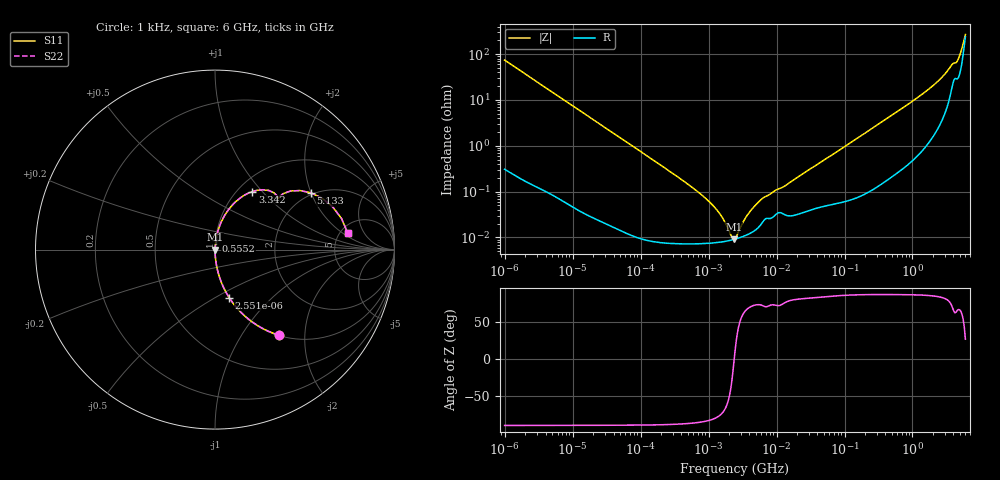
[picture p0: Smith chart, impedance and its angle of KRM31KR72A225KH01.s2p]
!Murata Part Number: KRM31KR72A225KH01
!These Parameters are Measured in Series Mode Connection
!Data Generated on Jan 08, 2026
!  o--ll--o
!Port1  Port2
!  o------o
!Operation Temp=25[degC], DC Bias Voltage=0[V]
!Freq. Start=1000[Hz] Stop=6[GHz] 401[Steps]
# Hz S RI R 50
!Freq.(Hz) S11(Real) S11(Imag) S21(Real) S21(Imag) S12(Real) S12(Imag) S22(Real) S22(Imag)
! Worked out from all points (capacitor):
!   401 points, 1 kHz to 6 GHz, reference 50 ohm
!   read as one part in series: C = 2.15 uF near 1.081 kHz
!   lowest |Z| = 9.07 mohm at 2.356 MHz (marker M1)
!   series resonance near 2.384 MHz, so ESL is about 2.1 nH
!   S11 on the Smith chart (normalised r, x): 1 kHz: 1.01, -1.48; 2.551 kHz: 1.00, -0.58; 555.2 MHz: 1.00, +0.10; 3.342 GHz: 1.17, +0.89; 5.133 GHz: 1.94, +1.99; 6 GHz: 5.78, +2.44
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1000  0.3549 -0.4764  0.6451 0.4764  0.6451 0.4764  0.3549 -0.4764
2551  0.0792 -0.2677  0.9208 0.2677  0.9208 0.2677  0.0792 -0.2677
5567  0.0183 -0.1312  0.9817 0.1312  0.9817 0.1312  0.0183 -0.1312
13657  0.00333 -0.0545  0.9967 0.0545  0.9967 0.0545  0.00333 -0.0545
186501  9.38e-05 -0.00401  0.9999 0.00401  0.9999 0.00401  9.38e-05 -0.00401
556098  7.39e-05 -0.00128  0.9999 0.00128  0.9999 0.00128  7.39e-05 -0.00128
1038191  7.51e-05 -0.000586  0.9999 0.000586  0.9999 0.000586  7.51e-05 -0.000586
1474979  7.89e-05 -0.000313  0.9999 0.000313  0.9999 0.000313  7.89e-05 -0.000313
2095531  8.66e-05 -8.08e-05  0.9999 8.08e-05  0.9999 8.08e-05  8.66e-05 -8.08e-05
2355756  9.04e-05 -7.4e-06  0.9999 7.4e-06  0.9999 7.4e-06  9.04e-05 -7.4e-06
2449490  9.18e-05 1.69e-05  0.9999 -1.69e-05  0.9999 -1.69e-05  9.18e-05 1.69e-05
3762485  0.000116 0.000292  0.9999 -0.000292  0.9999 -0.000292  0.000116 0.000292
5779283  0.000184 0.000621  0.9998 -0.000621  0.9998 -0.000621  0.000184 0.000621
3.345153e7  0.000418 0.00329  0.9996 -0.00329  0.9996 -0.00329  0.000418 0.00329
4.568318e8  0.00371 0.0423  0.9963 -0.0423  0.9963 -0.0423  0.00371 0.0423
5.552431e8  0.00499 0.0513  0.995 -0.0513  0.995 -0.0513  0.00499 0.0513
1.935242e9  0.0499 0.1836  0.9501 -0.1836  0.9501 -0.1836  0.0499 0.1836
2.644224e9  0.1063 0.2581  0.8937 -0.2581  0.8937 -0.2581  0.1063 0.2581
3.341724e9  0.2086 0.3236  0.7914 -0.3236  0.7914 -0.3236  0.2086 0.3236
4.565976e9  0.3789 0.3111  0.6211 -0.3111  0.6211 -0.3111  0.3789 0.3111
5.132982e9  0.5341 0.3163  0.4659 -0.3163  0.4659 -0.3163  0.5341 0.3163
6e9  0.7388 0.0942  0.2612 -0.0942  0.2612 -0.0942  0.7388 0.0942
